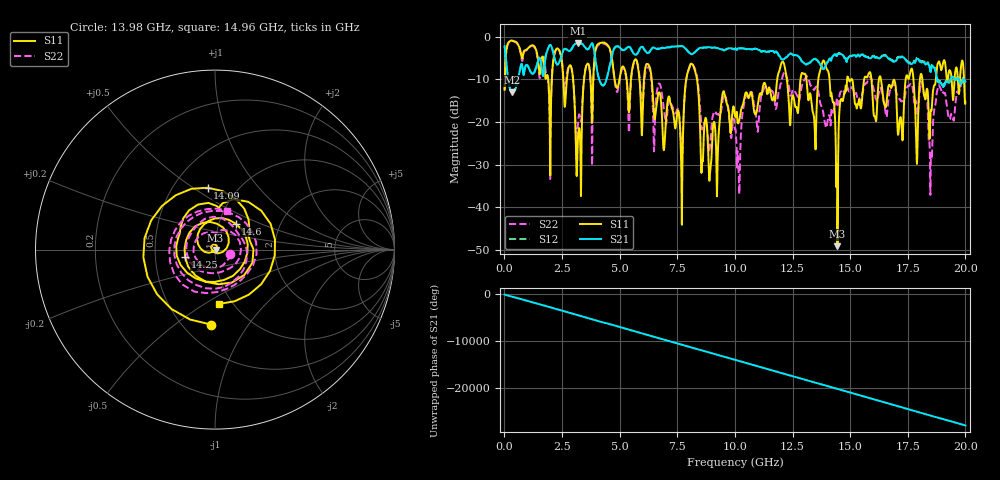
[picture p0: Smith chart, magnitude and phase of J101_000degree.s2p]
!Keysight Technologies,N5222A,MY51421036,A.10.65.16
!Date: Friday, March 31, 2023 14:49:02
!Correction: S11(Full 2 Port(1,2))
!S21(Full 2 Port(1,2))
!S12(Full 2 Port(1,2))
!S22(Full 2 Port(1,2))
!S2P File: Measurements: S11, S21, S12, S22:
# Hz S  dB  R 50
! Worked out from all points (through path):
!   2000 points, 10 MHz to 20 GHz, reference 50 ohm
!   highest |S21| = -1.56 dB at 3.18 GHz (marker M1); lowest = -13.0 dB at 320 MHz (marker M2)
!   group delay of S21, straight-line fit = 3.9 ns
!   lowest |S11| = -49.1 dB at 14.45 GHz (marker M3), VSWR 1.01, Z = 50.3 - j0.188 ohm
!   |S11| at or under -10 dB: 6.391 GHz to 7.886 GHz (1.495 GHz wide, 20.9 % of centre); 8.357 GHz to 11.84 GHz (3.48 GHz wide, 34.5 % of centre); 16.34 GHz to 17.41 GHz (1.071 GHz wide, 6.35 % of centre)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
!   |S22| runs from -37.1 to -0.9 dB; largest |S21 - S12| = 0.023
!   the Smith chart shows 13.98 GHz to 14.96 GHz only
!   S11 on the Smith chart (normalised r, x): 13.98 GHz: 0.68, -0.69; 14.09 GHz: 0.73, +0.57; 14.25 GHz: 0.71, -0.06; 14.6 GHz: 1.20, +0.36; 14.96 GHz: 0.87, -0.58
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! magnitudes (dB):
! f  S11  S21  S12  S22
! 10 MHz  -12.4  -2.2  -2.2  -12.4
! 320 MHz  -0.9  -13.0  -13.0  -0.9
! 2.87 GHz  -6.8  -3.2  -3.2  -6.8
! 3.18 GHz  -25.0  -1.6  -1.5  -21.5
! 3.35 GHz  -24.2  -1.6  -1.6  -18.6
! 4.15 GHz  -1.5  -10.5  -10.5  -1.7
! 6.68 GHz  -13.2  -2.9  -2.8  -11.2
! 7.68 GHz  -33.2  -2.2  -2.1  -29.2
! 8.17 GHz  -6.5  -4.0  -4.0  -6.5
! 8.92 GHz  -32.1  -2.5  -2.4  -25.5
! 10.01 GHz  -18.7  -2.8  -2.8  -21.6
! 13.34 GHz  -16.1  -5.6  -5.5  -11.7
! 13.98 GHz  -7.6  -6.3  -6.2  -21.2
! 14.09 GHz  -9.2  -5.3  -5.2  -18.5
! 14.25 GHz  -15.3  -4.6  -4.5  -17.8
! 14.45 GHz  -49.1  -4.1  -4.0  -15.8
! 14.6 GHz  -14.7  -4.1  -4.0  -12.8
! 14.96 GHz  -10.3  -4.7  -4.6  -12.8
! 16.67 GHz  -11.4  -5.2  -5.0  -14.1
! 18.14 GHz  -10.3  -6.0  -5.7  -11.4
! 18.49 GHz  -17.8  -8.3  -8.1  -31.6
! 20 GHz  -15.2  -10.5  -10.0  -10.6
